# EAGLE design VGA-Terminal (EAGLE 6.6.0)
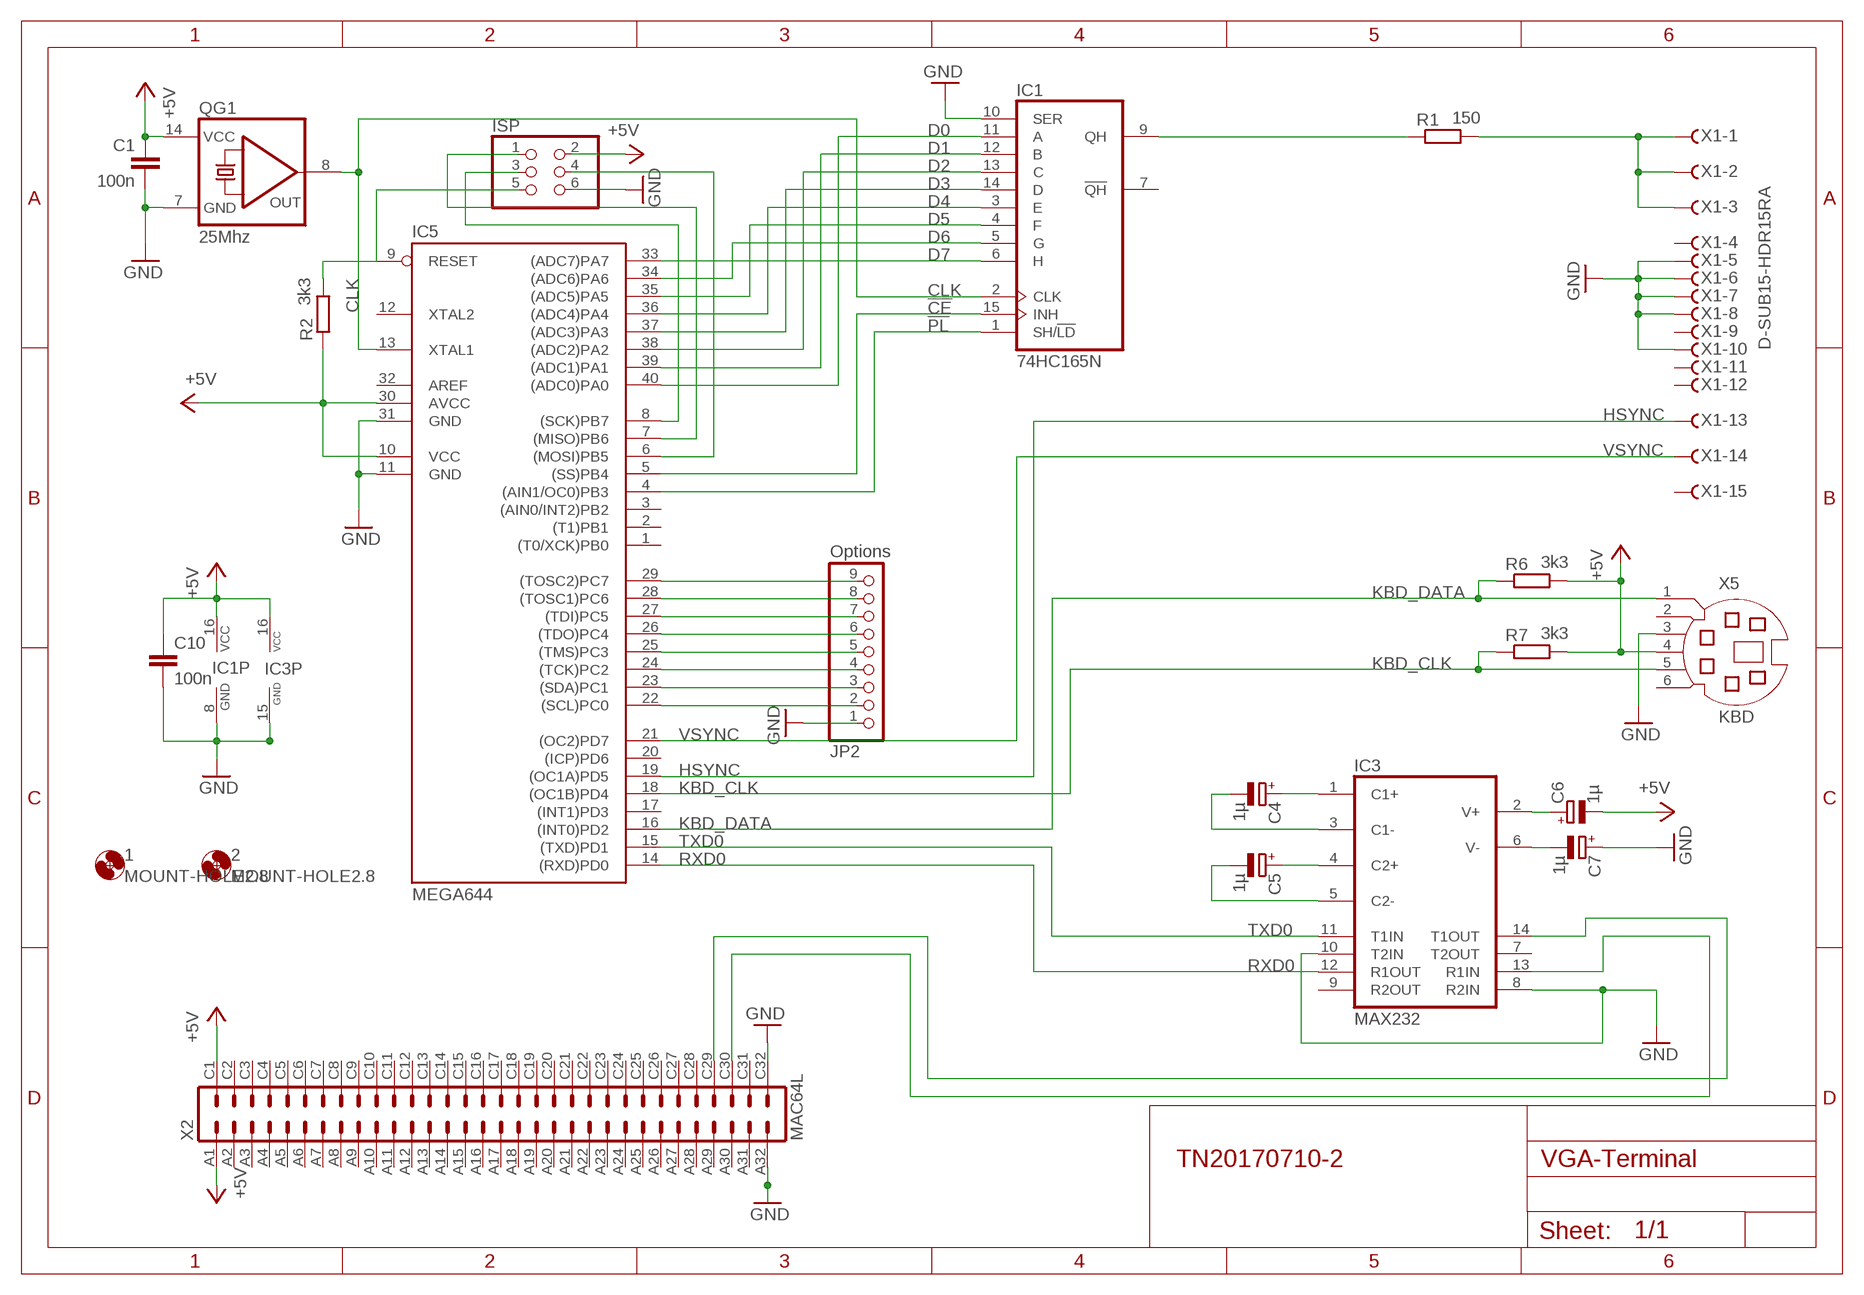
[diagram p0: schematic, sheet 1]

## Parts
1  MOUNT-HOLE2.8  [2,8]
2  MOUNT-HOLE2.8  [2,8]
C1  100n  C-EU025-025X050  [C025-025X050]
C4  1µ  CPOL-EUE2,5-6E  [E2,5-6E]
C5  1µ  CPOL-EUE5-5  [E5-5]
C6  1µ  CPOL-EUE5-5  [E5-5]
C7  1µ  CPOL-EUE2,5-6E  [E2,5-6E]
C10  100n  C-EU025-025X050  [C025-025X050]
IC1  74HC165N  [DIL16]
IC3  MAX232  [DIL16]
IC5  MEGA644  MEGA16-P  [DIL40]
ISP  PINHD-2X3  [2X03]
JP2  Options  PINHD-1X9  [1X09]
QG1  25Mhz  QG5860  [DIL14S]
R1  150  R-EU_0204/7  [0204/7]
R2  3k3  R-EU_0204/7  [0204/7]
R6  3k3  R-EU_0204/7  [0204/7]
R7  3k3  R-EU_0204/7  [0204/7]
X1  D-SUB15-HDR15RA  [HDR15RA]
X2  MAC64L  [MAC64L]
X5  KBD  MD06SS  [MDIN06SS]

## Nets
!CE: IC1.15(INH) IC5.5((SS)PB4)
!PL: IC1.1(SH/!LD) IC5.4((AIN1/OC0)PB3)
+5V: C1.1 C6.- C10.1 IC1.16(VCC) IC3.16(VCC) IC5.10(VCC) IC5.30(AVCC) ISP.2 QG1.14(VCC) R2.1 R6.2 R7.2 X2.A1 X2.C1 X5.4
CLK: IC1.2(CLK) IC5.13(XTAL1) QG1.8(OUT)
D0: IC1.11(A) IC5.40((ADC0)PA0)
D1: IC1.12(B) IC5.39((ADC1)PA1)
D2: IC1.13(C) IC5.38((ADC2)PA2)
D3: IC1.14(D) IC5.37((ADC3)PA3)
D4: IC1.3(E) IC5.36((ADC4)PA4)
D5: IC1.4(F) IC5.35((ADC5)PA5)
D6: IC1.5(G) IC5.34((ADC6)PA6)
D7: IC1.6(H) IC5.33((ADC7)PA7)
GND: C1.2 C7.+ C10.2 IC1.8(GND) IC1.10(SER) IC3.8(R2IN) IC3.10(T2IN) IC3.15(GND) IC5.11(GND) IC5.31(GND) ISP.6 JP2.1 QG1.7(GND) X1.5 X1.6 X1.7 X1.8 X1.10 X2.A32 X2.C32 X5.3
HSYNC: IC5.19((OC1A)PD5) X1.13
KBD_CLK: IC5.18((OC1B)PD4) R7.1 X5.5
KBD_DATA: IC5.16((INT0)PD2) R6.1 X5.1
MISO: IC5.7((MISO)PB6) ISP.1
MOSI: IC5.6((MOSI)PB5) ISP.4
N$2: IC1.9(QH) R1.1
N$3: IC5.29((TOSC2)PC7) JP2.9
N$6: C4.+ IC3.1(C1+)
N$7: C4.- IC3.3(C1-)
N$8: C5.+ IC3.4(C2+)
N$10: IC5.28((TOSC1)PC6) JP2.8
N$11: C5.- IC3.5(C2-)
N$12: C7.- IC3.6(V-)
N$13: C6.+ IC3.2(V+)
N$14: IC5.27((TDI)PC5) JP2.7
N$15: IC5.26((TDO)PC4) JP2.6
N$16: IC5.25((TMS)PC3) JP2.5
N$17: IC5.24((TCK)PC2) JP2.4
N$24: IC5.23((SDA)PC1) JP2.3
N$25: IC5.22((SCL)PC0) JP2.2
RESET: IC5.9(RESET) ISP.5 R2.2
RGB: R1.2 X1.1 X1.2 X1.3
RS232-RX: IC3.13(R1IN) X2.C30
RS232-TX: IC3.14(T1OUT) X2.C29
RXD0: IC3.12(R1OUT) IC5.14((RXD)PD0)
SCK: IC5.8((SCK)PB7) ISP.3
TXD0: IC3.11(T1IN) IC5.15((TXD)PD1)
VSYNC: IC5.21((OC2)PD7) X1.14
Unconnected: IC1.7(!QH) IC3.7(T2OUT) IC3.9(R2OUT) IC5.1((T0/XCK)PB0) IC5.2((T1)PB1) IC5.3((AIN0/INT2)PB2) IC5.12(XTAL2) IC5.17((INT1)PD3) IC5.20((ICP)PD6) IC5.32(AREF) X1.4 X1.9 X1.11 X1.12 X1.15 X2.A2 X2.A3 X2.A4 X2.A5 X2.A6 X2.A7 X2.A8 X2.A9 X2.A10 X2.A11 X2.A12 X2.A13 X2.A14 X2.A15 X2.A16 X2.A17 X2.A18 X2.A19 X2.A20 X2.A21 X2.A22 X2.A23 X2.A24 X2.A25 X2.A26 X2.A27 X2.A28 X2.A29 X2.A30 X2.A31 X2.C2 X2.C3 X2.C4 X2.C5 X2.C6 X2.C7 X2.C8 X2.C9 X2.C10 X2.C11 X2.C12 X2.C13 X2.C14 X2.C15 X2.C16 X2.C17 X2.C18 X2.C19 X2.C20 X2.C21 X2.C22 X2.C23 X2.C24 X2.C25 X2.C26 X2.C27 X2.C28 X2.C31 X5.2 X5.6

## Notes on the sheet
- TN20170710-2

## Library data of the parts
1 2 = holes:MOUNT-HOLE: MOUNTING HOLE with drill center marker
C1 C10 = rcl:C-EU: CAPACITOR, European symbol
C4-C7 = rcl:CPOL-EU: POLARIZED CAPACITOR, European symbol
IC1 = 74xx-eu:74*165: 8-bit parallel load SHIFT REGISTER
IC3 = maxim:MAX232: RS232 TRANSEIVER
IC5 = atmel:MEGA16-P: MICROCONTROLLER 16 Kbytes FLASH 1 kbytes SRAM 512 bytes EEPROM USART 8-channel 10 bit ADC Source: avr.lbr
ISP = pinhead:PINHD-2X3: PIN HEADER
JP2 = pinhead_sqr:PINHD-1X9: PIN HEADER
QG1 = crystal:QG5860: CRYSTAL RESONATOR
R1 R2 R6 R7 = rcl:R-EU_: RESISTOR, European symbol
X1 = con-thomas-betts:D-SUB15-: D-Subminiatur Connector Source: Electronioc Interconnects European Edition 1998
X2 = con-vg:MAC64L: CONNECTOR male, 64 pins, block, type C, rows AC, grid 5.08 mm
X5 = con-yamaichi:MD06SS: YAMAICHI CONNECTOR

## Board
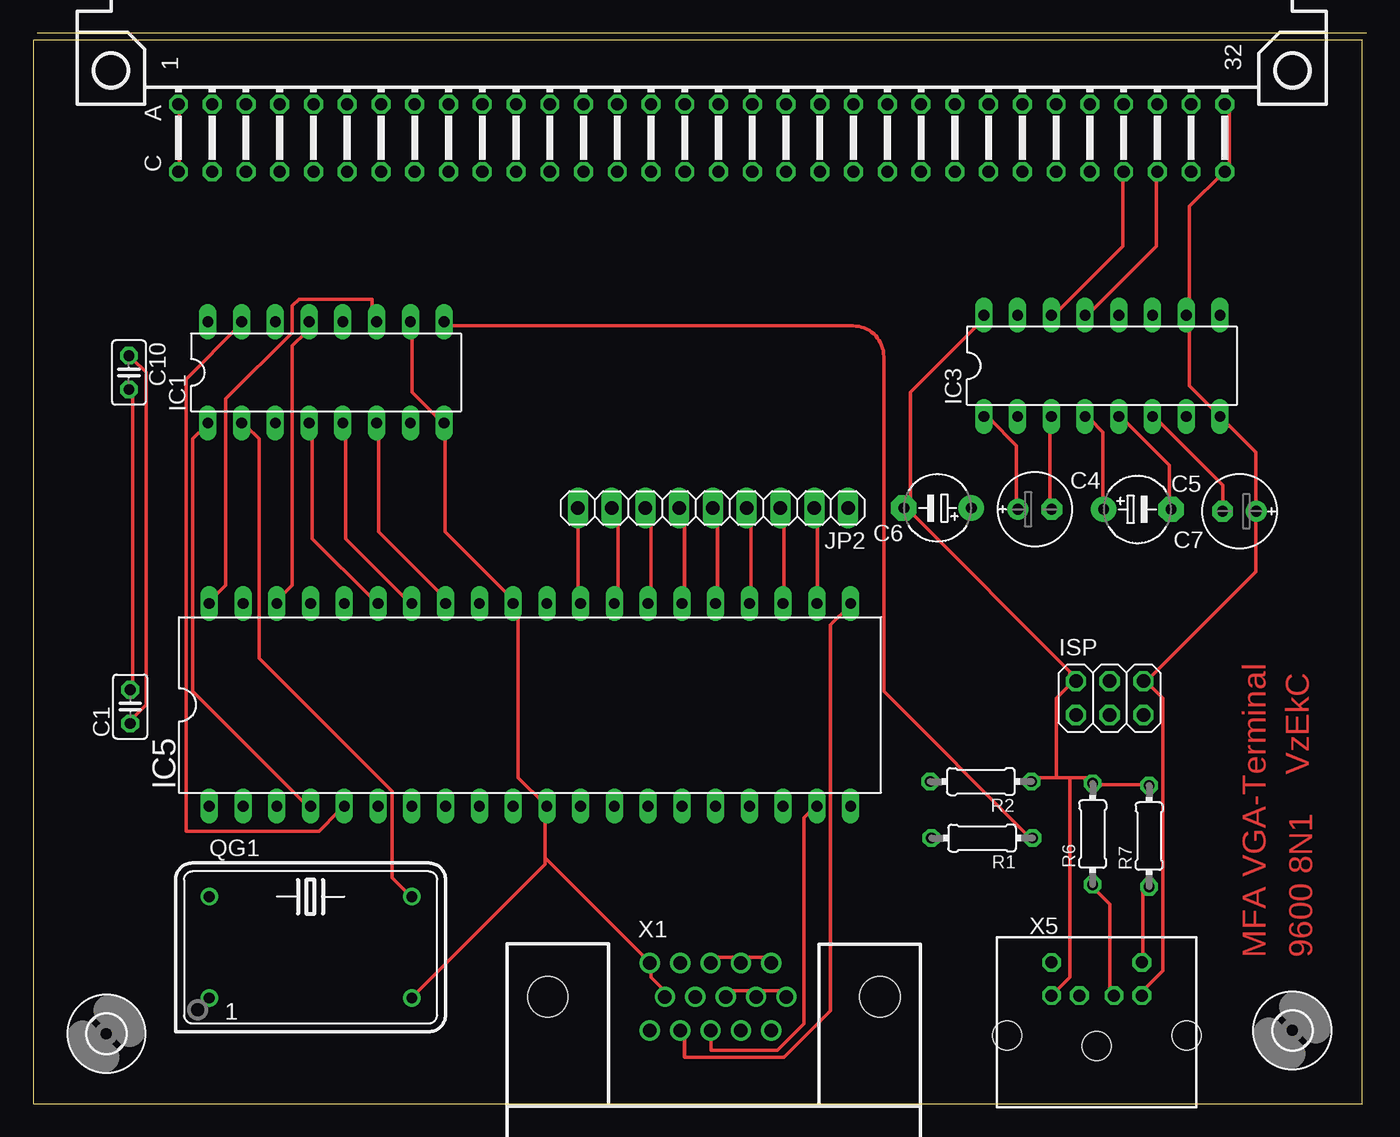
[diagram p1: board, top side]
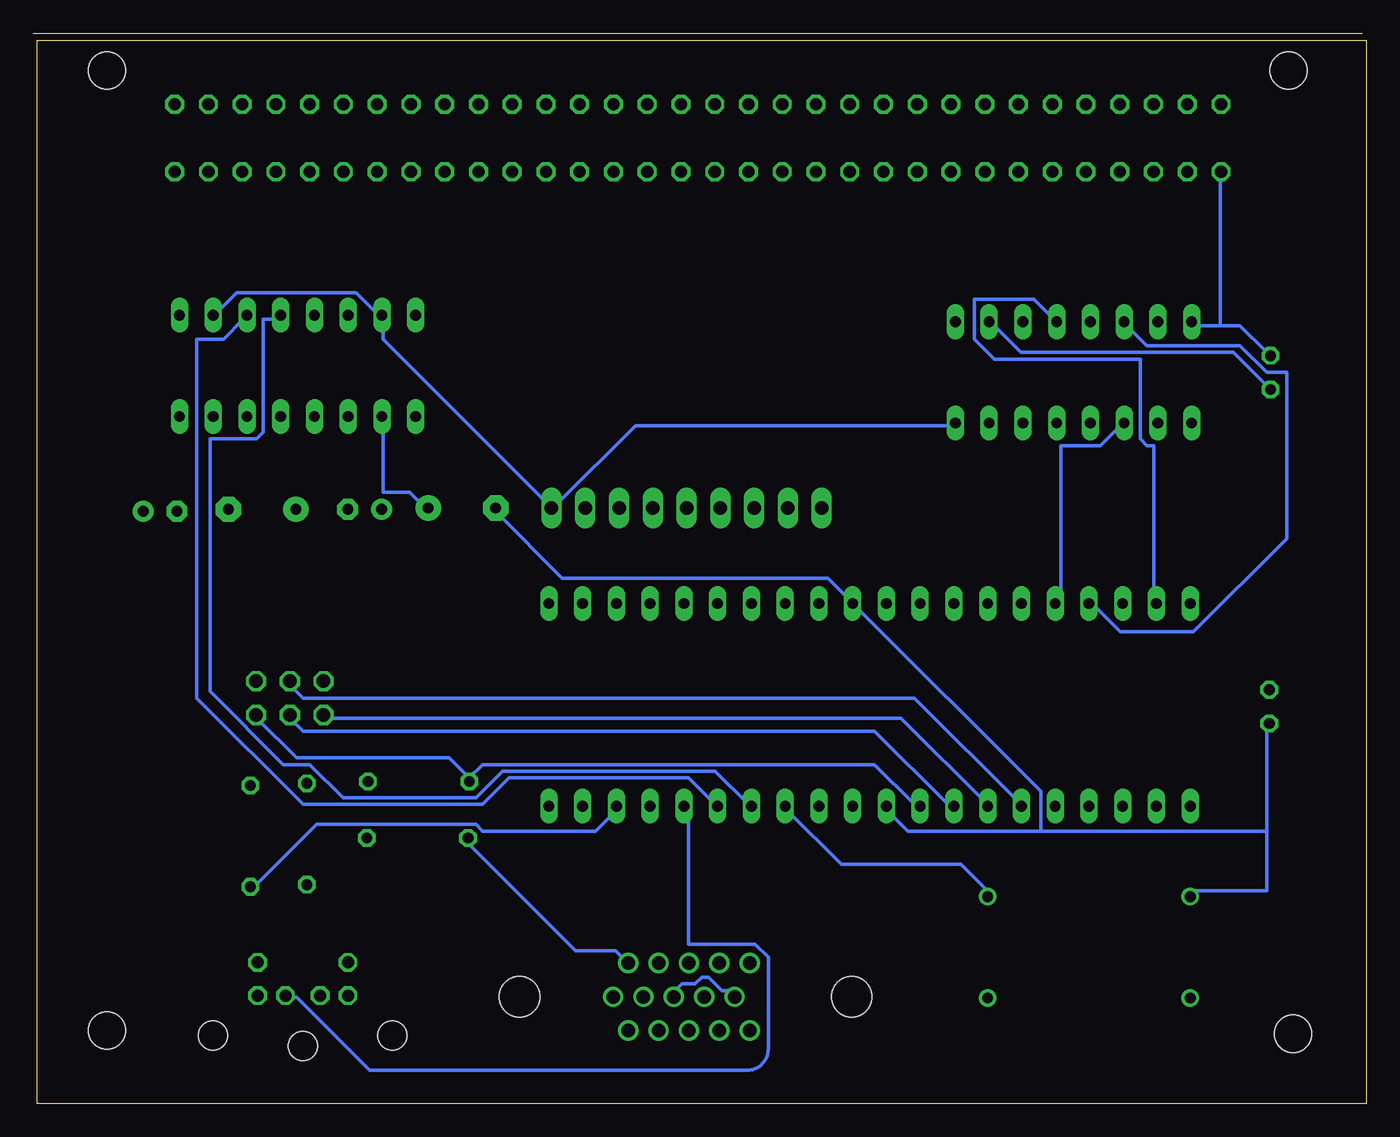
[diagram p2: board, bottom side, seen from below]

Size 100.31 x 80.51 mm. Coordinates in mm from the lower left corner, seen from the top.
Outline: 0,0 100,0 100,80 0,80 0,0
Copper layers (1*16): Top 0.035mm / dielectric 1.5mm / Bottom 0.035mm
Design rules "default": minimum track width 10mil, minimum drill 24mil, track to track 8mil, track to pad 8mil, pad to pad 8mil, via to via 8mil, smd to smd 8mil, copper to edge 40mil, drill to drill 8mil, minimum pad ring 10mil, minimum via ring 8mil, stop-mask expansion 4mil, vias tented up to drill 0mil, thermal gap 10mil

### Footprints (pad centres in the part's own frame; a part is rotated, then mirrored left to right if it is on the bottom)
2,8 = hole 2.8: 0,0
C025-025X050 = drill 0.813 octagon: 1 -1.27,0; 2 1.27,0
E2,5-6E = drill 0.813 pad 1.575: + -1.27,0 | drill 0.813 pad 1.575 octagon: - 1.27,0
E5-5 = drill 0.813 pad 1.905: + -2.54,0 | drill 0.813 pad 1.905 octagon: - 2.54,0
DIL16 = drill 0.813 long: 1 -8.89,-3.81; 2 -6.35,-3.81; 3 -3.81,-3.81; 4 -1.27,-3.81; 5 1.27,-3.81; 6 3.81,-3.81; 7 6.35,-3.81; 8 8.89,-3.81; 9 8.89,3.81; 10 6.35,3.81; 11 3.81,3.81; 12 1.27,3.81; 13 -1.27,3.81; 14 -3.81,3.81; 15 -6.35,3.81; 16 -8.89,3.81
DIL40 = drill 0.813 long: 1 -24.13,-7.62; 2 -21.59,-7.62; 3 -19.05,-7.62; 4 -16.51,-7.62; 5 -13.97,-7.62; 6 -11.43,-7.62; 7 -8.89,-7.62; 8 -6.35,-7.62; 9 -3.81,-7.62; 10 -1.27,-7.62; 11 1.27,-7.62; 12 3.81,-7.62; 13 6.35,-7.62; 14 8.89,-7.62; 15 11.43,-7.62; 16 13.97,-7.62; 17 16.51,-7.62; 18 19.05,-7.62; 19 21.59,-7.62; 20 24.13,-7.62; 21 24.13,7.62; 22 21.59,7.62; 23 19.05,7.62; 24 16.51,7.62; 25 13.97,7.62; 26 11.43,7.62; 27 8.89,7.62; 28 6.35,7.62; 29 3.81,7.62; 30 1.27,7.62; 31 -1.27,7.62; 32 -3.81,7.62; 33 -6.35,7.62; 34 -8.89,7.62; 35 -11.43,7.62; 36 -13.97,7.62; 37 -16.51,7.62; 38 -19.05,7.62; 39 -21.59,7.62; 40 -24.13,7.62
2X03 = drill 1.016 octagon: 1 -2.54,-1.27; 2 -2.54,1.27; 3 0,-1.27; 4 0,1.27; 5 2.54,-1.27; 6 2.54,1.27
1X09 = drill 1.016 long: 1 -10.16,0; 2 -7.62,0; 3 -5.08,0; 4 -2.54,0; 5 0,0; 6 2.54,0; 7 5.08,0; 8 7.62,0; 9 10.16,0
DIL14S = drill 0.813: 1 -7.62,-3.81; 7 7.62,-3.81; 8 7.62,3.81; 14 -7.62,3.81
0204/7 = drill 0.813 octagon: 1 -3.81,0; 2 3.81,0
HDR15RA = drill 1.016: 1 4.318,2.54; 2 2.032,2.54; 3 -0.254,2.54; 4 -2.54,2.54; 5 -4.826,2.54; 6 5.461,0; 7 3.175,0; 8 0.889,0; 9 -1.397,0; 10 -3.683,0; 11 4.318,-2.54; 12 2.032,-2.54; 13 -0.254,-2.54; 14 -2.54,-2.54; 15 -4.826,-2.54 | hole 3.048: -12.497,0; 12.497,0
MAC64L = drill 0.914 octagon: A1 -2.54,39.37; A2 -2.54,36.83; A3 -2.54,34.29; A4 -2.54,31.75; A5 -2.54,29.21; A6 -2.54,26.67; A7 -2.54,24.13; A8 -2.54,21.59; A9 -2.54,19.05; A10 -2.54,16.51; A11 -2.54,13.97; A12 -2.54,11.43; A13 -2.54,8.89; A14 -2.54,6.35; A15 -2.54,3.81; A16 -2.54,1.27; A17 -2.54,-1.27; A18 -2.54,-3.81; A19 -2.54,-6.35; A20 -2.54,-8.89; A21 -2.54,-11.43; A22 -2.54,-13.97; A23 -2.54,-16.51; A24 -2.54,-19.05; A25 -2.54,-21.59; A26 -2.54,-24.13; A27 -2.54,-26.67; A28 -2.54,-29.21; A29 -2.54,-31.75; A30 -2.54,-34.29; A31 -2.54,-36.83; A32 -2.54,-39.37; C1 -7.62,39.37; C2 -7.62,36.83; C3 -7.62,34.29; C4 -7.62,31.75; C5 -7.62,29.21; C6 -7.62,26.67; C7 -7.62,24.13; C8 -7.62,21.59; C9 -7.62,19.05; C10 -7.62,16.51; C11 -7.62,13.97; C12 -7.62,11.43; C13 -7.62,8.89; C14 -7.62,6.35; C15 -7.62,3.81; C16 -7.62,1.27; C17 -7.62,-1.27; C18 -7.62,-3.81; C19 -7.62,-6.35; C20 -7.62,-8.89; C21 -7.62,-11.43; C22 -7.62,-13.97; C23 -7.62,-16.51; C24 -7.62,-19.05; C25 -7.62,-21.59; C26 -7.62,-24.13; C27 -7.62,-26.67; C28 -7.62,-29.21; C29 -7.62,-31.75; C30 -7.62,-34.29; C31 -7.62,-36.83; C32 -7.62,-39.37 | hole 2.794: 0,44.45; 0,-44.45
MDIN06SS = drill 0.9 octagon: 1 1.3,8.5; 2 -1.3,8.5; 3 3.4,8.5; 4 -3.4,8.5; 5 3.4,11; 6 -3.4,11 | hole 2.2: -6.75,5.5; 0,4.7; 6.75,5.5

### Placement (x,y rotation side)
1  5.5,5.25 0 top
2  94.75,5.5 0 top
C1  7.3,29.86 90 top
C4  75.37,44.7 0 top
C5  83.09,44.7 0 top
C6  68.05,44.8 180 top
C7  90.77,44.55 180 top
C10  7.2,54.99 270 top
IC1  22.03,55 0 top
IC3  80.42,55.5 0 top
IC5  37.38,29.99 0 top
ISP  81,30.5 0 top
JP2  51.15,44.8 180 top
QG1  20.87,11.75 0 top
R1  71.4,19.97 180 top
R2  71.31,24.22 180 top
R6  79.72,20.28 90 top
R7  83.97,20.12 90 top
X1  51.22,8.03 0 top
X2  50.3,77.72 90 top
X5  80.03,-0.38 0 top

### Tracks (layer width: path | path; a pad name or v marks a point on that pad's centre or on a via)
!CE
  Top 0.254: IC5.5 23,22 21.5,20.5 11.5,20.5 11.5,54.5 15.5,58.5 IC1.15
!PL
  Top 0.254: IC5.4 20.5,22.5 12,31 12,50 13,51 IC1.1
+5V
  Top 0.254: IC3.16 71.5,59 66,53.5 66,45 C6.- 66,44.5 78,32.5 78,32 ISP.2 78,31.5 77,30.5 77,24.5 | R7.2 83.5,24 80,24 R6.2 79.5,24.5 78,24.5 | 78,24.5 77,24.5 | 77,24.5 75.5,24.5 R2.1 | 78,24.5 78,9.5 77,8.5 X5.4 | X2.C1 11,70.5 11,75 X2.A1 | C10.1 7.5,56 8.5,55 8.5,30 7.5,29 C1.1
  Bottom 0.254: 11,58.5 13,58.5 IC1.16 | 11,58.5 9.5,58.5 7.5,56.5 C10.1 | 11,58.5 11,70 X2.C1 | 7.5,20.5 7.5,16 13,16 QG1.14 | 7.5,20.5 7.5,28.5 C1.1 | 7.5,20.5 24.5,20.5 | 24.5,20.5 34.5,20.5 36,22 IC5.10 | 24.5,20.5 24.5,23.5 38.5,37.5 IC5.30 39,38 40.5,39.5 60.5,39.5 65.5,44.5 C6.-
CLK
  Top 0.254: IC1.2 16,51 17,50 17,33.5 27,23.5 27,17 28,16 QG1.8
  Bottom 0.254: QG1.8 28.5,16 30.5,18 39.5,18 43.5,22 IC5.13
D0
  Top 0.254: IC5.40 13.5,38 14.5,39 14.5,53 19.5,58 19.5,60 20,60.5 25.5,60.5 25.5,59 IC1.11
D1
  Bottom 0.254: IC5.39 16,38 16,49.5 16.5,49.5 17,50 17,56 28,56 29.5,57.5 29.5,60.5 25,60.5 23.5,59 IC1.12
D2
  Top 0.254: IC5.38 18.5,38 19.5,39 19.5,57 20.5,58 20.5,58.5 IC1.13
D3
  Bottom 0.254: IC5.37 20.5,37.5 18.5,35.5 13,35.5 6,42.5 6,55 7.5,55 9.5,57 16.5,57 18,58.5 IC1.14
D4
  Bottom 0.254: IC5.36 23,38 23,49.5 20,49.5 18.5,51 IC1.3
D5
  Top 0.254: IC5.35 25.5,38 21,42.5 21,51 IC1.4
D6
  Top 0.254: IC5.34 28,38 23.5,42.5 23.5,51 IC1.5
D7
  Top 0.254: IC5.33 31,38 26,43 26,51 IC1.6
GND
  Top 0.254: X5.3 83.5,8.5 85,10 85,30.5 84,31.5 ISP.6 84,32 92,40 92,44.5 C7.+ 92,45 92,49 IC3.8 87,54 87,59 IC3.10 87,59.5 87,67.5 89.5,70 X2.C32 90,70.5 90,75 X2.A32 | X1.8 52.5,8.5 54,8.5 X1.7 54.5,8.5 56.5,8.5 X1.6 | X1.10 47.5,8.5 46.5,9.5 46.5,10.5 X1.5 46,11 38.5,18.5 | 38.5,18.5 38.5,22 IC5.11 38.5,22.5 36.5,24.5 36.5,37.5 IC5.31 36,38 31,43 31,51 IC1.8 30.5,51.5 28.5,53.5 28.5,58.5 IC1.10 | 38.5,18.5 38.5,18 28.5,8 QG1.7 | C1.2 7.5,31.5 7.5,53.5 C10.2
  Bottom 0.254: IC3.10 86.5,59.5 85,61 76,61 74.5,59.5 IC3.15 74,59 74,57.5 61.5,45 JP2.1 61,45 55,51 31,51 IC1.8 | X1.8 52,8.5 51.5,9 50.5,9 50,9.5 49.5,9.5 48.5,8.5 48,8.5 X1.10 | C10.2 7.5,54 10,56.5 26,56.5 28,58.5 IC1.10
HSYNC
  Top 0.254: IC5.19 58.5,22 58,21.5 58,6 56,4 51,4 51,5 X1.13
KBD_CLK
  Top 0.254: X5.5 83.5,11 83.5,16 R7.1
  Bottom 0.254: IC5.18 56.5,22 58,20.5 66.5,20.5 67,21 79,21 83.5,16.5 R7.1
KBD_DATA
  Top 0.254: R6.1 80,16 81,15 81,8.5 X5.1
  Bottom 0.254: IC5.16 51,22 51,12 46,12 45,11 45,4.1 arc90 46.6,2.5 75,2.5 80.5,8 81,8 X5.1
MISO
  Bottom 0.254: IC5.7 28.5,22.5 35,29 78,29 ISP.1
MOSI
  Bottom 0.254: IC5.6 26,22.5 34,30.5 80,30.5 81,31.5 ISP.4
N$2
  Top 0.254: IC1.9 31,58.5 61.7,58.5 arc-90 64,56.2 64,31 75,20 R1.1
N$3
  Top 0.254: IC5.29 41,38 41,44.5 JP2.9
N$6
  Top 0.254: IC3.1 72,51.5 74,49.5 74,45 C4.+
N$7
  Top 0.254: IC3.3 76.5,51.5 76.5,45 C4.-
N$8
  Top 0.254: IC3.4 79.5,51.5 80.5,50.5 80.5,45 C5.+
N$10
  Top 0.254: IC5.28 44,38 44,44.5 JP2.8
N$11
  Top 0.254: IC3.5 82,51.5 85.5,48 85.5,45 C5.-
N$12
  Top 0.254: C7.- 89.5,46.5 84.5,51.5 IC3.6
N$13
  Bottom 0.254: IC3.2 74,51.5 74,46 72,46 71,45 C6.+
N$14
  Top 0.254: IC5.27 46.5,38 46.5,44.5 JP2.7
N$15
  Top 0.254: IC5.26 49,38 49,44.5 JP2.6
N$16
  Top 0.254: IC5.25 51.5,38 51.5,44.5 JP2.5
N$17
  Top 0.254: IC5.24 54,38 54,44.5 JP2.4
N$24
  Top 0.254: IC5.23 56.5,38 56.5,44.5 JP2.3
N$25
  Top 0.254: IC5.22 59,38 59,44.5 JP2.2
RESET
  Bottom 0.254: 67.5,24.5 66.5,25.5 37,25.5 34,22.5 IC5.9 | 67.5,24.5 69,26 80.5,26 83.5,29 ISP.5 | 67.5,24.5 R2.2
RGB
  Top 0.254: X1.3 51,11 53,11 X1.2 53.5,11 55.5,11 X1.1
  Bottom 0.254: R1.2 67.5,19.5 59.5,11.5 56.5,11.5 56,11 X1.1
RS232-RX
  Top 0.254: IC3.13 79.5,59.5 84.5,64.5 84.5,70 X2.C30
RS232-TX
  Top 0.254: IC3.14 77,59.5 82,64.5 82,70 X2.C29
RXD0
  Bottom 0.254: IC5.14 46.5,22.5 49,25 65,25 67,23 77,23 79.5,25.5 81.5,25.5 87,31 87,50 83.5,50 83,50.5 83,59 82,59 IC3.12
SCK
  Bottom 0.254: IC5.8 31.5,22.5 37,28 80,28 81,29 ISP.3
TXD0
  Bottom 0.254: IC5.15 49,22.5 51,24.5 64.5,24.5 66.5,22.5 80,22.5 88,30.5 88,57.5 86,57.5 84.5,59 IC3.11
VSYNC
  Top 0.254: IC5.21 61.5,37.5 60,36 60,7 56.5,3.5 49,3.5 49,5 X1.14

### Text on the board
Top: VzEkC | MFA VGA-Terminal | 9600 8N1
